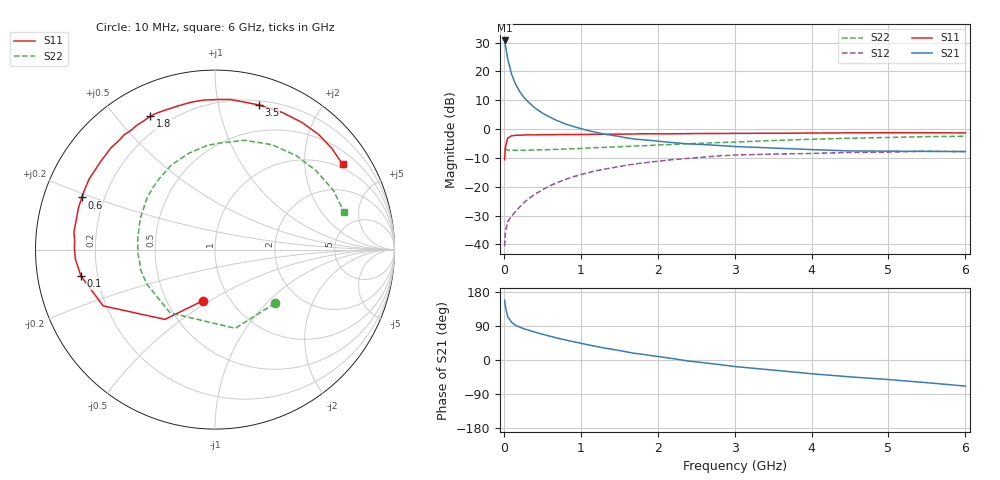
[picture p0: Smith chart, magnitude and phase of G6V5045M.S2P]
! SIEMENS Small Signal Semiconductors
! BFG193
! Si NPN RF Bipolar Junction Transistor in SOT223
! VCE = 0.5 V  IC = 45 mA
! Common Emitter S-Parameters:  August  1996
# GHz  S  MA  R  50
!  f  S11  S21  S12  S22
! GHz  MAG  ANG  MAG  ANG  MAG  ANG  MAG  ANG
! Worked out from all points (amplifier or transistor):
!   36 points, 10 MHz to 6 GHz, reference 50 ohm
!   highest |S21| = 30.7 dB at 10 MHz (marker M1)
!   |S21| within 3 dB of that: start of sweep to 29.07 MHz
!   unconditionally stable (mu >= 1): start of sweep to 13.26 MHz; 150 MHz to end of sweep
!   at 250 MHz: K = 1.18, MAG = 16.0 dB, |S12| = -25.9 dB
!   at 1.4 GHz: K = 1.24, MAG = 2.7 dB, |S12| = -13.5 dB
!   at 6 GHz: K = 1.08, MAG = -1.7 dB, |S12| = -7.8 dB
!   S11 on the Smith chart (normalised r, x): 10 MHz: 0.75, -0.47; 100 MHz: 0.14, -0.10; 600 MHz: 0.12, +0.19; 1.8 GHz: 0.13, +0.62; 3.5 GHz: 0.24, +1.32; 6 GHz: 0.87, +3.07
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0.01  0.2926 -103.2  34.33 157.7  0.0093 67.7  0.4479 -42.0
0.02  0.4787 -125.7  28.75 141.0  0.0162 55.6  0.4528 -75.6
0.05  0.6977 -153.3  16.49 114.6  0.0246 43.1  0.4325 -125.4
0.1  0.761 -168.8  8.987 99.7  0.0309 44.4  0.4257 -153.4
0.15  0.7791 -175.9  6.073 92.0  0.037 48.8  0.4292 -164.7
0.2  0.7833 179.7  4.609 87.2  0.0436 53.2  0.4251 -171.1
0.25  0.7838 176.2  3.692 83.2  0.0509 55.6  0.43 -176.2
0.3  0.7921 172.9  3.098 79.9  0.0584 57.4  0.4289 -179.5
0.4  0.7906 167.6  2.341 73.8  0.0735 58.6  0.4338 174.2
0.5  0.7955 163.1  1.896 68.1  0.0881 58.2  0.436 169.1
0.6  0.7968 158.6  1.599 62.8  0.1039 57.2  0.4392 165.0
0.7  0.8005 154.3  1.386 57.5  0.1186 55.6  0.4446 161.0
0.8  0.8039 150.5  1.226 53.0  0.1334 53.6  0.4509 157.1
1.1  0.8058 139.2  0.937 40.0  0.1753 47.1  0.4678 146.4
1.3  0.8095 131.8  0.818 31.8  0.2009 42.2  0.4804 139.2
1.8  0.8266 115.8  0.652 15.3  0.2573 29.2  0.5116 123.4
2.2  0.8264 104.5  0.58 3.6  0.2946 18.2  0.5394 111.4
2.8  0.8365 88.7  0.518 -12.0  0.3422 2.9  0.5829 94.0
3.5  0.8422 73.1  0.468 -26.6  0.3678 -15.3  0.6309 74.8
4.5  0.8583 55.6  0.417 -44.5  0.3929 -33.9  0.6924 49.1
5.5  0.8614 41.0  0.409 -59.8  0.4129 -54.9  0.7373 26.7
6  0.855 33.8  0.406 -68.9  0.4069 -66.8  0.7496 16.1
